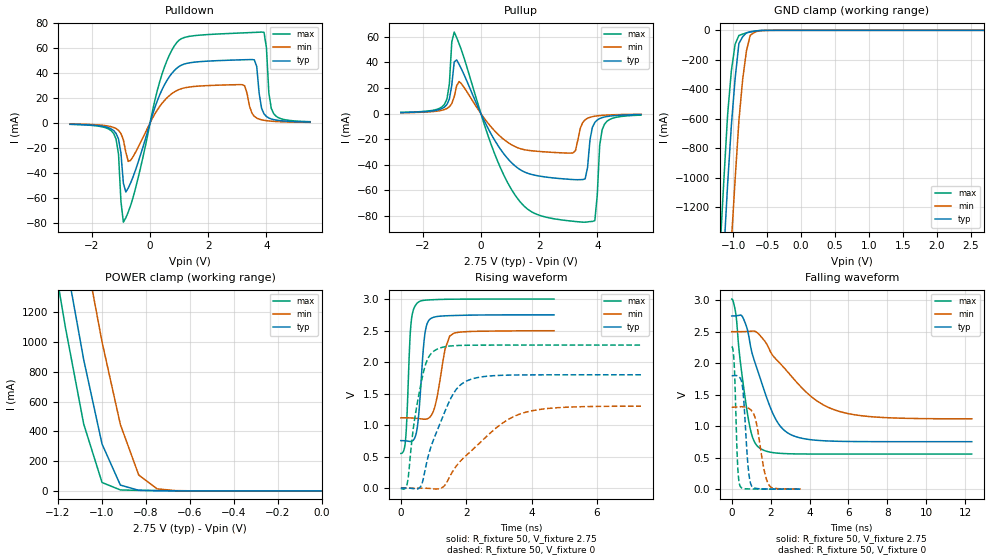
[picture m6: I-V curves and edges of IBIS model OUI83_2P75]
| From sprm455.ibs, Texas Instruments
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|   Model Cell OUI83_2P75
|OUI83_2P75
[Model]   OUI83_2P75
Model_type   3-state
Polarity   Non-Inverting
Enable   Active-Low
Cref =  15.0000pF
Rref =  100.000M
Vref =  0V
Vmeas =  1.375
C_comp   1.8817p   1.799p   2.0762p
[Temperature Range]   25   125   -40
[Voltage Range]   2.75   2.5   3
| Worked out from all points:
|   slope of the pulldown table from 0 to 0.412 V, typ, clamps not added: 15.5 ohm
|   slope of the pullup table from 0 to 0.412 V, typ, clamps not added: 22.4 ohm
|   GND clamp passes 1 mA (typ) near -0.58 V on its own axis
|   POWER clamp passes 1 mA (typ) near -0.68 V on its own axis
|   rising waveform, R_fixture 50, V_fixture 2.75: 20-80 % time 169ps typ, 278ps min, 118ps max; typ from 0.755 V to 2.75 V
|   rising waveform, R_fixture 50, V_fixture 0: 20-80 % time 771ps typ, 1.55ns min, 402ps max; typ from 0 V to 1.8 V
|   falling waveform, R_fixture 50, V_fixture 2.75: 20-80 % time 1.27ns typ, 2.49ns min, 602ps max; typ from 2.75 V to 0.754 V
|   falling waveform, R_fixture 50, V_fixture 0: 20-80 % time 228ps typ, 423ps min, 142ps max; typ from 1.8 V to 0.001 V
[POWER_clamp]
|   voltage   I(typ)   I(min)   I(max)
-2.75V    16.79A     17.52A     16.39A
-1.194V   1.811A     2.617A     1.344A
-1.139V   1.338A     2.134A     883.6mA
-1.083V   881.6mA    1.66A      449.5mA
-1.056V   692.7mA    1.44A      318.6mA
-1.028V   503.9mA    1.22A      187.6mA
-1V       315mA      1.001A     56.65mA
-916.7mV  39.29mA    445.8mA    6.508mA
-833.3mV  4.304mA    107.2mA    3.736mA
-750mV    1.762mA    13.87mA    2.231mA
-666.7mV  894.8uA    2.186mA    1.083mA
0V        28.08pA    4.523nA    346.4fA
[Pulldown]
|   voltage   I(typ)   I(min)   I(max)
-2.75V    -974.3uA   -755.5uA   -1.079mA
-1.25V    -6.071mA   -3.58mA    -8.439mA
-1.083V   -12.86mA   -5.876mA   -24.99mA
-916.7mV  -48.13mA   -13.44mA   -79.32mA
-666.7mV  -47.87mA   -29.87mA   -65.9mA
333.3mV   22.59mA    13.28mA    33.12mA
1.083V    46.33mA    27.47mA    67.49mA
3.167V    50.55mA    30.63mA    72.03mA
3.583V    50.52mA    5.33mA     72.45mA
3.917V    7.298mA    2.134mA    72.52mA
4.25V     2.705mA    1.306mA    7.401mA
5.5V      771.4uA    522.6uA    1.048mA
[Pullup]
|   voltage   I(typ)   I(min)   I(max)
-2.75V    781.9uA    636.2uA    897.4uA
-1.25V    5.061mA    3.14mA     7.246mA
-1.083V   11.26mA    5.325mA    22.87mA
-916.7mV  40.27mA    13.02mA    63.53mA
-750mV    38.45mA    24.96mA    54.5mA
1.167V    -40.69mA   -25.69mA   -63.3mA
3.167V    -51.47mA   -30.68mA   -84mA
3.583V    -50.93mA   -4.86mA    -84.72mA
3.917V    -6.885mA   -2.059mA   -83.47mA
4.083V    -3.89mA    -1.583mA   -24.7mA
4.25V     -2.678mA   -1.282mA   -8.239mA
5.5V      -781.8uA   -522.3uA   -1.214mA
[GND_clamp]
|   voltage   I(typ)   I(min)   I(max)
-2.75V    -16.99A    -17.78A    -16.55A
-1.194V   -1.993A    -2.86A     -1.488A
-1.139V   -1.513A    -2.371A    -1.02A
-1.083V   -1.048A    -1.89A     -574.4mA
-1.028V   -645.5mA   -1.437A    -273.6mA
-972.2mV  -326.2mA   -1.012A    -93.77mA
-916.7mV  -89.52mA   -614.2mA   -34.96mA
-861.1mV  -43.42mA   -333.5mA   -25.67mA
-805.6mV  -16.84mA   -140.1mA   -17.63mA
-750mV    -9.779mA   -34.06mA   -10.85mA
-638.9mV  -3.1mA     -5.425mA   -2.719mA
2.694V    25.79pA    429.6nA    216.1fA
[Ramp]
| variable   typ   min   max
dV/dt_f   1.206237/1.270251n   0.8367443/2.496662n   1.477095/0.6018424n
dV/dt_r   1.088388/0.7734999n  0.7892445/1.562474n   1.371625/0.4023864n
R_load = 50
[Rising Waveform]
R_fixture = 50
V_fixture = 2.75
V_fixture_min = 2.5
V_fixture_max = 3
|   time   V(typ)   V(min)   V(max)
0s        754.5mV    1.115V     549.9mV
156ps     749.5mV    1.116V     846.9mV
306ps     741.5mV    1.114V     2.588V
498ps     945.5mV    1.107V     2.935V
708ps     2.33V      1.094V     2.98V
900ps     2.686V     1.133V     2.987V
1.062ns   2.719V     1.337V     2.991V
1.356ns   2.734V     2.21V      2.996V
1.494ns   2.737V     2.413V     2.997V
4.686ns   2.75V      2.497V     3V
[Rising Waveform]
R_fixture = 50
V_fixture = 0
V_fixture_min = 0
V_fixture_max = 0
|   time   V(typ)   V(min)   V(max)
0s        241.8uV    -62.87uV   -4.191mV
192ps     849.9uV    137.8uV    64.31mV
390ps     -8.084mV   391.9uV    983.1mV
618ps     36.89mV    594.6uV    1.664V
804ps     438.1mV    -2.083mV   2.031V
1.062ns   851.4mV    -12.85mV   2.192V
1.614ns   1.506V     289.9mV    2.26V
2.172ns   1.732V     600.9mV    2.268V
3.828ns   1.797V     1.206V     2.27V
7.344ns   1.799V     1.3V       2.27V
[Falling Waveform]
R_fixture = 50
V_fixture = 2.75
V_fixture_min = 2.5
V_fixture_max = 3
|   time   V(typ)   V(min)   V(max)
0s        2.749V     2.5V       3.018V
222ps     2.752V     2.499V     2.765V
444ps     2.764V     2.5V       2.025V
888ps     2.414V     2.504V     1.059V
1.146ns   2.058V     2.509V     765.1mV
1.47ns    1.756V     2.435V     645.4mV
2.406ns   1.037V     2.022V     570.7mV
3.408ns   822.9mV    1.674V     559.4mV
6.06ns    756.9mV    1.195V     557.4mV
12.34ns   753.7mV    1.117V     557.4mV
[Falling Waveform]
R_fixture = 50
V_fixture = 0
V_fixture_min = 0
V_fixture_max = 0
|   time   V(typ)   V(min)   V(max)
0s        1.8V       1.302V     2.265V
120ps     1.803V     1.302V     2.03V
288ps     1.799V     1.306V     493.9mV
426ps     1.767V     1.309V     53.3mV
588ps     1.536V     1.308V     11.03mV
834ps     385.4mV    1.29V      4.456mV
1.008ns   59.63mV    1.251V     3.226mV
1.26ns    11.71mV    1.063V     2.136mV
1.926ns   2.809mV    59.94mV    739.7uV
3.552ns   688.6uV    2.514mV    97.85uV
